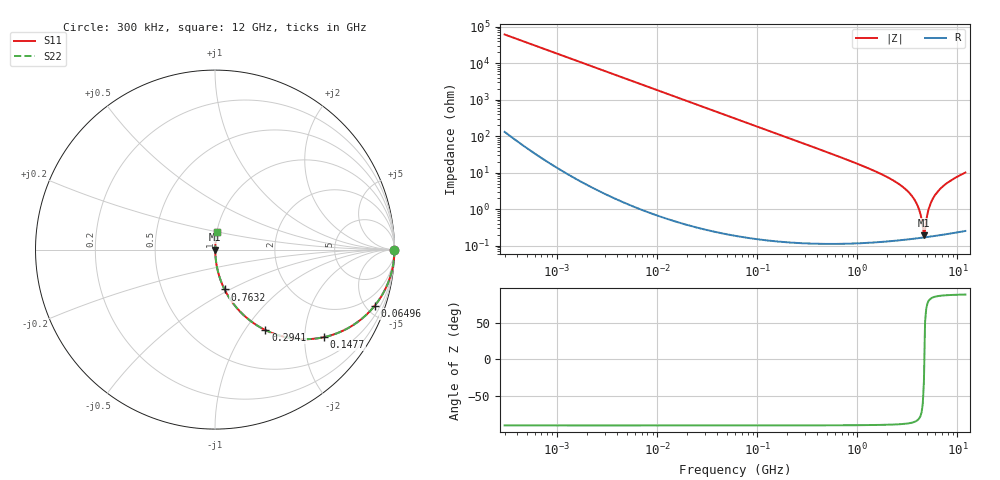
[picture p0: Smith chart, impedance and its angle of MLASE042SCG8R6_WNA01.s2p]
! MLASE042SCG8R6_WNA01  S-PARAMETER MODEL  ( General Type )
! Model Generated by TAIYO YUDEN Corporation (http://www.ty-top.com)
! Version 1.0
! TAIYO YUDEN Control No. 130801
! Copyright(c) 2013 TAIYO YUDEN CO.,LTD. All Rights Reserved.
! Product Description (link to TY-COMPAS)
! https://ds.yuden.co.jp/TYCOMPAS/or/detail?pn=MLASE042SCG8R6BWNA01&u=M
! Products Name : Multilayer Ceramic Capacitors
! Characteristics :
!  Capacitance : 8.6 pF , Rated Voltage : 16V , TCC : CG / C0G
!  Case Size : 0.4 x 0.2 / 0.016 x 0.008 [mm/inch] , Thickness : 0.2 / 0.008 [mm/inch]
!  (Conditions: Temperature = 25 degC , DC Bias Current/Voltage = 0A / 0V)
! External Node Assignments :
!  1  o---| |---o  2
! GND o---------o GND
! Frequency Range : 0.3MHz  -  12000MHz  [ 401 STEP ]
# MHz S RI R 50
! Freq[MHz].  S11 Real  S11 Imag  S21 Real  S21 Imag  S12 Real  S12 Imag  S22 Real  S22 Imag
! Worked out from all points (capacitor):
!   401 points, 300 kHz to 12 GHz, reference 50 ohm
!   read as one part in series: C = 8.64 pF near 316.3 kHz
!   lowest |Z| = 194 mohm at 4.624 GHz (marker M1)
!   series resonance near 4.663 GHz, so ESL is about 130 pH
!   S11 on the Smith chart (normalised r, x): 300 kHz: open; 64.96 MHz: 1.00, -5.67; 147.7 MHz: 1.00, -2.49; 294.1 MHz: 1.00, -1.25; 763.2 MHz: 1.00, -0.47; 12 GHz: 1.01, +0.20
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0.3  1 -0.00163  6.13e-06 0.00163  6.13e-06 0.00163  1 -0.00163
1.769972  0.9999 -0.0096  9.73e-05 0.0096  9.73e-05 0.0096  0.9999 -0.0096
10.44266  0.9968 -0.0565  0.00322 0.0565  0.00322 0.0565  0.9968 -0.0565
26.39317  0.9798 -0.1403  0.0202 0.1403  0.0202 0.1403  0.9798 -0.1403
60  0.904 -0.2943  0.096 0.2943  0.096 0.2943  0.904 -0.2943
64.96309  0.8893 -0.3135  0.1107 0.3135  0.1107 0.3135  0.8893 -0.3135
147.6816  0.6083 -0.4876  0.3917 0.4876  0.3917 0.4876  0.6083 -0.4876
294.0765  0.2807 -0.4484  0.7193 0.4484  0.7193 0.4484  0.2807 -0.4484
353.9943  0.2118 -0.4075  0.7882 0.4075  0.7882 0.4075  0.2118 -0.4075
763.2128  0.0533 -0.2222  0.9467 0.2222  0.9467 0.2222  0.0533 -0.2222
2088.533  0.00626 -0.0701  0.9937 0.0701  0.9937 0.0701  0.00626 -0.0701
2870.14  0.00302 -0.0398  0.997 0.0398  0.997 0.0398  0.00302 -0.0398
3547.679  0.00201 -0.022  0.998 0.022  0.998 0.022  0.00201 -0.022
4050.141  0.00173 -0.0113  0.9983 0.0113  0.9983 0.0113  0.00173 -0.0113
4502.883  0.00167 -0.00294  0.9983 0.00294  0.9983 0.00294  0.00167 -0.00294
4623.766  0.00168 -0.000967  0.9983 0.000967  0.9983 0.000967  0.00168 -0.000967
4875.354  0.00173 0.0045  0.9983 -0.0045  0.9983 -0.0045  0.00173 0.0045
5140.631  0.00184 0.00973  0.9982 -0.00973  0.9982 -0.00973  0.00184 0.00973
5420.343  0.00199 0.0146  0.998 -0.0146  0.998 -0.0146  0.00199 0.0146
6188.031  0.00263 0.0275  0.9974 -0.0275  0.9974 -0.0275  0.00263 0.0275
8064.993  0.00504 0.0541  0.995 -0.0541  0.995 -0.0541  0.00504 0.0541
12000  0.0126 0.0995  0.9874 -0.0995  0.9874 -0.0995  0.0126 0.0995
